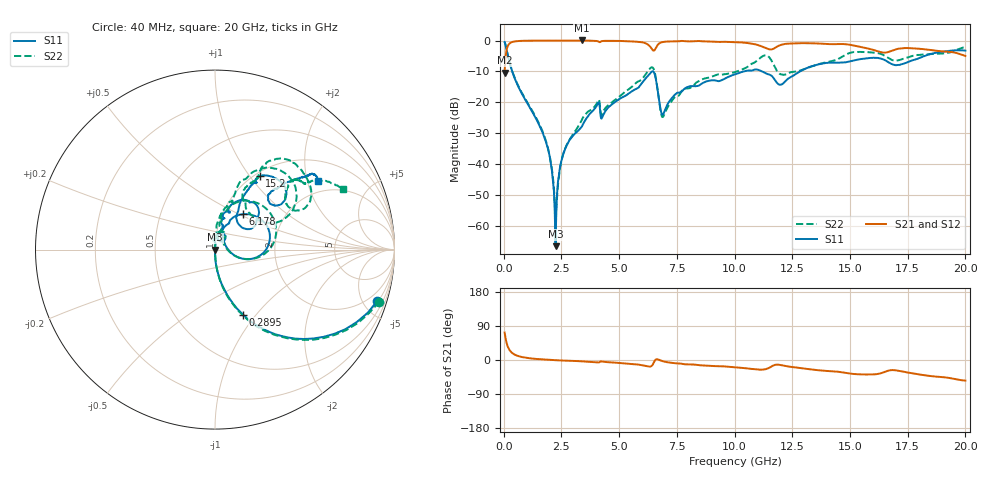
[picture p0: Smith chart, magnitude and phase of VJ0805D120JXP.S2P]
! VJ0805D120JXP
! DATE 10/29/2021  12:02
! CAPACITORS MOUNTED IN SERIES ON 25 MIL THICK MICROSTRIP SUBSTRATE
# GHz  S  MA  R  50.00
!  FREQ  S11M  S11A  S21M  S21A  S12M  S12A  S22M  S22A
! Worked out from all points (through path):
!   1601 points, 40 MHz to 20 GHz, reference 50 ohm
!   highest |S21| = 0.04 dB at 3.383 GHz (marker M1); lowest = -10.4 dB at 40 MHz (marker M2)
!   group delay of S21, straight-line fit = 7.61 ps
!   lowest |S11| = -66.6 dB at 2.248 GHz (marker M3), VSWR 1.00, Z = 50 + j0.0132 ohm
!   |S11| at or under -10 dB: 369.4 MHz to 6.424 GHz (6.055 GHz wide, 178 % of centre); 6.48 GHz to 10.4 GHz (3.92 GHz wide, 46.5 % of centre); 11.19 GHz to 12.83 GHz (1.645 GHz wide, 13.7 % of centre)
!   |S22| runs from -57.9 to -0.4 dB; largest |S21 - S12| = 0.0076
!   S11 on the Smith chart (normalised r, x): 40 MHz: 1.11, -6.29; 289.5 MHz: 1.00, -0.86; 6.178 GHz: 1.24, +0.52; 15.2 GHz: 1.05, +1.12; 20 GHz: 1.61, +2.32
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0.04  0.9482 -17.5  0.3003 72.4  0.2996 72.3  0.9604 -17.7
0.2895  0.3948 -66.8  0.9182 23.3  0.9179 23.2  0.3991 -67.0
1.823925  0.02333 -89.3  0.9987 0.9  0.9995 0.9  0.02407 -86.0
2.023525  0.01134 -83.8  0.9982 0.2  0.999 0.1  0.01163 -82.0
2.248075  0.0004656 16.4  0.9985 -0.5  0.9987 -0.6  0.001456 -25.6
2.622325  0.01574 83.5  0.9985 -1.5  0.9988 -1.6  0.01613 86.7
3.370825  0.03975 90.3  1.005 -3.5  1.005 -3.6  0.05038 99.5
3.3833  0.04029 90.6  1.005 -3.5  1.005 -3.7  0.05171 99.7
4.044475  0.08994 75.6  0.9836 -6.2  0.9849 -6.3  0.09801 79.8
4.293975  0.05989 73.9  0.9861 -4.5  0.9872 -4.6  0.06831 78.5
6.1777  0.2505 52.0  0.8944 -16.2  0.8948 -16.4  0.2939 64.4
6.4771  0.3169 15.6  0.6898 -9.9  0.691 -10.1  0.3579 18.0
6.70165  0.1297 -18.4  0.8772 1.1  0.8776 1.1  0.129 -18.2
6.913725  0.06484 35.8  0.9523 -3.5  0.9533 -3.6  0.05896 36.7
7.79945  0.1619 77.1  0.9836 -11.0  0.9834 -11.1  0.1658 76.0
10.02  0.2836 67.2  0.9436 -19.0  0.9447 -19.2  0.309 70.5
11.47958  0.2834 35.4  0.7244 -21.3  0.7249 -21.6  0.5477 34.0
12.05343  0.1955 49.6  0.8608 -13.8  0.8614 -14.0  0.2811 41.2
13.35083  0.3847 60.9  0.9052 -25.1  0.9042 -25.3  0.3823 64.0
15.19712  0.4799 58.8  0.8264 -37.1  0.8274 -37.5  0.6518 48.1
16.68165  0.4418 34.5  0.6552 -27.9  0.6558 -28.2  0.5163 25.0
20  0.6864 33.7  0.5638 -54.4  0.5625 -54.8  0.789 25.2
